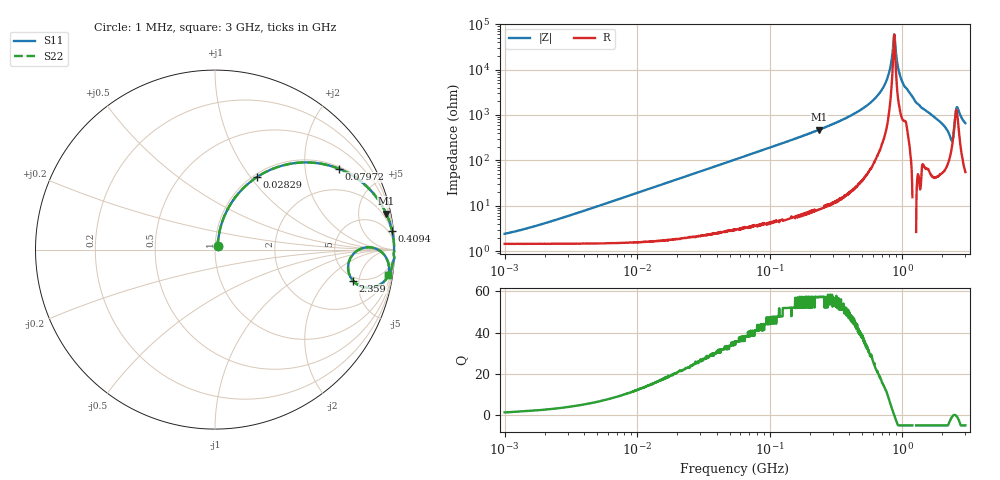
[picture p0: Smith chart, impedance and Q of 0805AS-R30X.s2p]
!s-Parameter Generated by FASTRON Sdn. Bhd.
!FASTRON P/N : 0805AS-R30X
!Keysight Technologies: E4991B_MY54100416_A.01.15
!Date: Fri Jan 09 15:12:22 2026
!Version  :Rev01  Tue Jan 13 16:04:05 2026
!Data & Calibration Information:
!Freq  S11  S21  S12  S22
!PortZ  Port1:50+j0  Port2:50+j0
!When reading reference impedance value at option line is always used.
! Remarks : This data is being provided solely for informational purposes.
# Hz S dB R 50
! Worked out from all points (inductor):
!   1601 points, 1 MHz to 3 GHz, reference 50 ohm
!   read as one part in series: L = 306 nH near 2.283 MHz
!   highest Q = 57.3 at 236.1 MHz (marker M1), where L = 318 nH
!   self-resonance near 871.6 MHz
!   S11 on the Smith chart (normalised r, x): 1 MHz: 1.03, +0.04; 28.29 MHz: 1.04, +1.08; 79.72 MHz: 1.08, +3.03; 409.4 MHz: 1, +19; 2.359 GHz: 4.54, -4.15; 3 GHz: 2, -13
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1000000  -32.50 51.9  -0.13 -1.1  -0.13 -1.1  -32.50 51.9
3804036  -22.70 74.5  -0.15 -4.1  -0.15 -4.1  -22.70 74.5
1.447069e7  -11.60 71.3  -0.46 -15.2  -0.46 -15.2  -11.60 71.3
2.829425e7  -6.60 59.9  -1.25 -27.8  -1.25 -27.8  -6.60 59.9
5.504702e7  -2.94 42.9  -3.33 -45.4  -3.33 -45.4  -2.94 42.9
7.971695e7  -1.67 33.0  -5.27 -55.6  -5.27 -55.6  -1.67 33.0
2.083556e8  -0.28 13.6  -12.60 -75.4  -12.60 -75.4  -0.28 13.6
2.361213e8  -0.22 11.9  -13.70 -77.1  -13.70 -77.1  -0.22 11.9
4.094372e8  -0.06 5.9  -19.80 -82.9  -19.80 -82.9  -0.06 5.9
6.423554e8  -0.02 2.2  -28.20 -85.1  -28.20 -85.1  -0.02 2.2
7.279565e8  -0.02 1.3  -32.70 -84.6  -32.70 -84.6  -0.02 1.3
7.925923e8  -0.01 0.7  -38.20 -82.2  -38.20 -82.2  -0.01 0.7
8.501091e8  -0.01 0.2  -48.70 -62.2  -48.70 -62.2  -0.01 0.2
8.760197e8  -0.01 -0.0  -55.10 19.7  -55.10 19.7  -0.01 -0.0
9.538021e8  -0.02 -0.7  -38.30 79.2  -38.30 79.2  -0.02 -0.7
1.0437e9  -0.04 -1.3  -32.60 78.6  -32.60 78.6  -0.04 -1.3
1.300759e9  -0.02 -3.2  -25.10 85.5  -25.10 85.5  -0.02 -3.2
2.01032e9  -0.22 -8.8  -16.30 76.4  -16.30 76.4  -0.22 -8.8
2.359433e9  -2.07 -12.7  -10.80 36.9  -10.80 36.9  -2.07 -12.7
2.492946e9  -1.15 0.7  -18.10 -5.1  -18.10 -5.1  -1.15 0.7
2.607784e9  -0.41 -2.7  -23.80 43.3  -23.80 43.3  -0.41 -2.7
3e9  -0.20 -8.5  -16.60 76.7  -16.60 76.7  -0.20 -8.5
